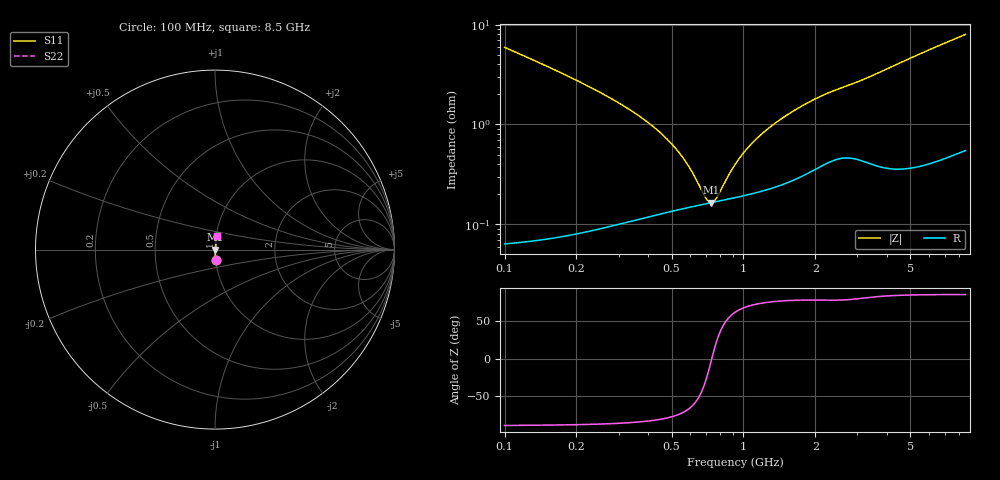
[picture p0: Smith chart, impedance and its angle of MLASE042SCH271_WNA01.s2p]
! MLASE042SCH271_WNA01  S-PARAMETER MODEL  ( General Type )
! Model Generated by TAIYO YUDEN Corporation (http://www.ty-top.com)
! Version 1.0
! TAIYO YUDEN Control No. 180301
! Copyright(c) 2018 TAIYO YUDEN CO.,LTD. All Rights Reserved.
! Product Description (link to TY-COMPAS)
! https://ds.yuden.co.jp/TYCOMPAS/or/detail?pn=MLASE042SCH271JWNA01&u=M
! Products Name : Multilayer Ceramic Capacitors
! Characteristics :
!  Capacitance : 270 pF , Rated Voltage : 16V , TCC : CH / C0H
!  Case Size : 0.4 x 0.2 / 0.016 x 0.008 [mm/inch] , Thickness : 0.2 / 0.008 [mm/inch]
!  (Conditions: Temperature = 25 degC , DC Bias Current/Voltage = 0A / 0V)
! External Node Assignments :
!  1  o---| |---o  2
! GND o---------o GND
! Frequency Range : 100MHz  -  8500MHz  [ 401 STEP ]
# MHz S RI R 50
! Freq[MHz].  S11 Real  S11 Imag  S21 Real  S21 Imag  S12 Real  S12 Imag  S22 Real  S22 Imag
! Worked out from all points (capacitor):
!   401 points, 100 MHz to 8.5 GHz, reference 50 ohm
!   read as one part in series: C = 265 pF near 102.2 MHz
!   lowest |Z| = 165 mohm at 730.2 MHz (marker M1)
!   series resonance near 736.7 MHz, so ESL is about 180 pH
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100  0.00411 -0.0588  0.9959 0.0588  0.9959 0.0588  0.00411 -0.0588
150.8243  0.00216 -0.038  0.9978 0.038  0.9978 0.038  0.00216 -0.038
212.8145  0.00148 -0.0256  0.9985 0.0256  0.9985 0.0256  0.00148 -0.0256
506.1018  0.0014 -0.00605  0.9986 0.00605  0.9986 0.00605  0.0014 -0.00605
584.7147  0.00148 -0.00365  0.9985 0.00365  0.9985 0.00365  0.00148 -0.00365
690.7124  0.0016 -0.00101  0.9984 0.00101  0.9984 0.00101  0.0016 -0.00101
714.1145  0.00163 -0.000485  0.9984 0.000485  0.9984 0.000485  0.00163 -0.000485
730.1548  0.00164 -0.000139  0.9984 0.000139  0.9984 0.000139  0.00164 -0.000139
746.5554  0.00166 0.000207  0.9983 -0.000207  0.9983 -0.000207  0.00166 0.000207
771.8496  0.00169 0.000725  0.9983 -0.000725  0.9983 -0.000725  0.00169 0.000725
862.518  0.00179 0.00245  0.9982 -0.00245  0.9982 -0.00245  0.00179 0.00245
921.9544  0.00186 0.0035  0.9981 -0.0035  0.9981 -0.0035  0.00186 0.0035
1041.762  0.002 0.00546  0.998 -0.00546  0.998 -0.00546  0.002 0.00546
1244.358  0.00228 0.00844  0.9977 -0.00844  0.9977 -0.00844  0.00228 0.00844
1502.954  0.00271 0.0119  0.9973 -0.0119  0.9973 -0.0119  0.00271 0.0119
1775.41  0.00329 0.0151  0.9967 -0.0151  0.9967 -0.0151  0.00329 0.0151
2097.259  0.00411 0.0185  0.9959 -0.0185  0.9959 -0.0185  0.00411 0.0185
2926.566  0.00516 0.0254  0.9948 -0.0254  0.9948 -0.0254  0.00516 0.0254
4317.005  0.00507 0.0388  0.9949 -0.0388  0.9949 -0.0388  0.00507 0.0388
5762.285  0.00672 0.0528  0.9933 -0.0528  0.9933 -0.0528  0.00672 0.0528
7116.102  0.00895 0.0655  0.9911 -0.0655  0.9911 -0.0655  0.00895 0.0655
8500  0.0116 0.0779  0.9884 -0.0779  0.9884 -0.0779  0.0116 0.0779
